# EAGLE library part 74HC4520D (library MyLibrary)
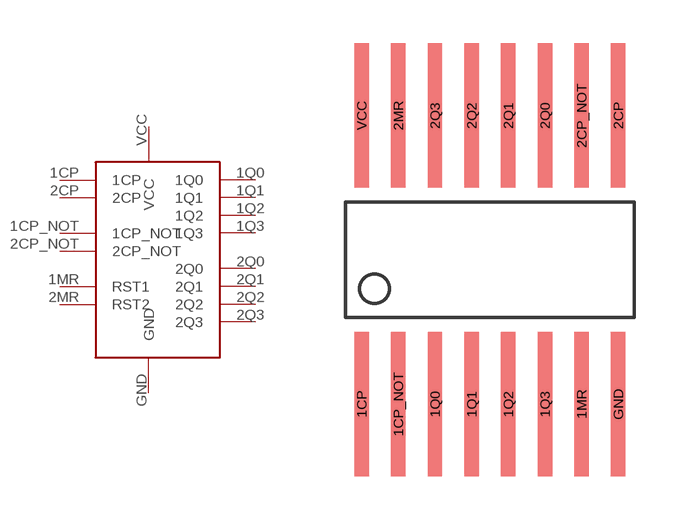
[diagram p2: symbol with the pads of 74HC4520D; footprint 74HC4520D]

Designator prefix -

## 74HC4520D  [74HC4520D]
1CP  1CP
1CP_NOT  1CP_NOT
1MR  RST1
1Q0  1Q0
1Q1  1Q1
1Q2  1Q2
1Q3  1Q3
2CP  2CP
2CP_NOT  2CP_NOT
2MR  RST2
2Q0  2Q0
2Q1  2Q1
2Q2  2Q2
2Q3  2Q3
GND  GND
VCC  VCC

## Footprint 74HC4520D (pad centres in mm)
smd 0.5 x 5: 1CP -4.445,-5; 1CP_NOT -3.175,-5; 1MR 3.175,-5; 1Q0 -1.905,-5; 1Q1 -0.635,-5; 1Q2 0.635,-5; 1Q3 1.905,-5; 2CP 4.445,5; 2CP_NOT 3.175,5; 2MR -3.175,5; 2Q0 1.905,5; 2Q1 0.635,5; 2Q2 -0.635,5; 2Q3 -1.905,5; GND 4.445,-5; VCC -4.445,5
